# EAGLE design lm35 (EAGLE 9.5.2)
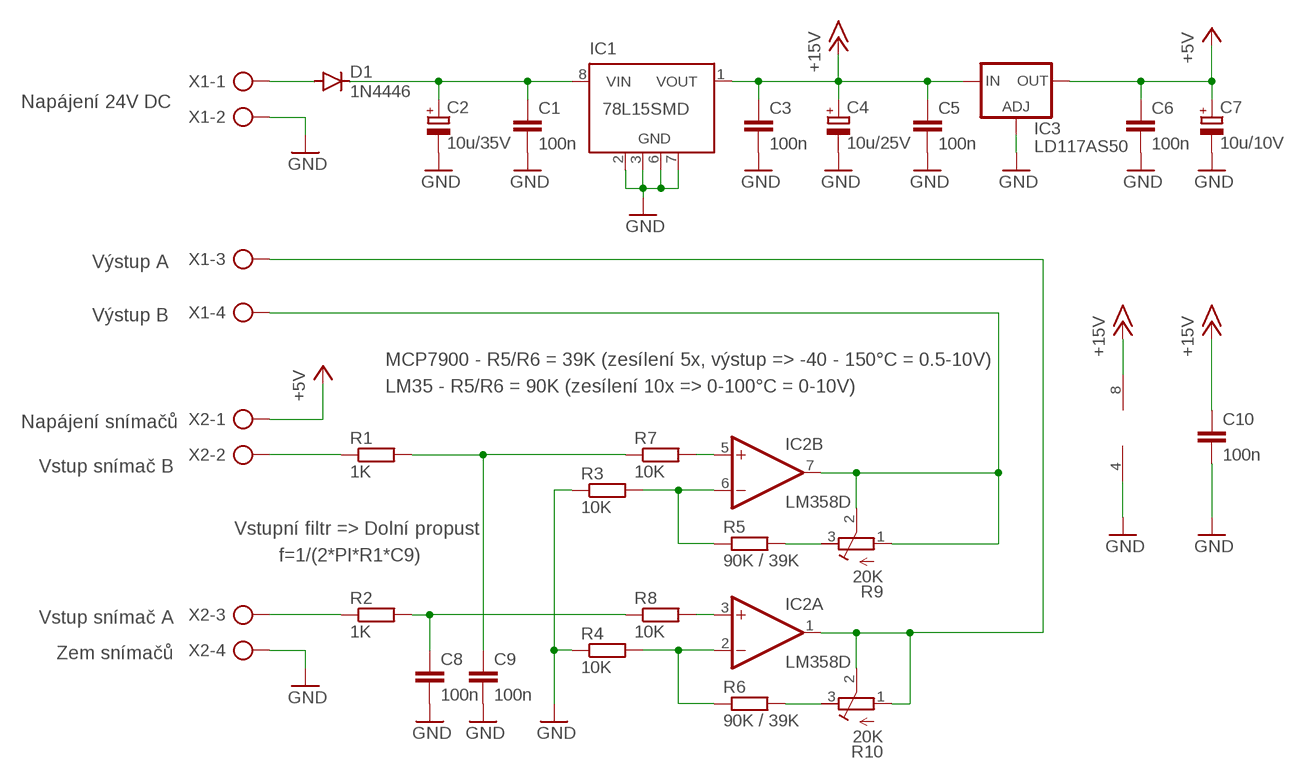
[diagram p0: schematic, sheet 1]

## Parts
C1  100n  C-EUC1206K  [C1206K]
C2  10u/35V  CPOL-EUE2.5-6  [E2,5-6]
C3  100n  C-EUC1206K  [C1206K]
C4  10u/25V  CPOL-EUE2.5-6  [E2,5-6]
C5  100n  C-EUC1206K  [C1206K]
C6  100n  C-EUC1206K  [C1206K]
C7  10u/10V  CPOL-EUE2.5-6  [E2,5-6]
C8  100n  C-EUC1206K  [C1206K]
C9  100n  C-EUC1206K  [C1206K]
C10  100n  C-EUC1206K  [C1206K]
D1  1N4446  [DO35-10]
IC1  78L15SMD  [SO08]
IC2  LM358D  [SO08]
IC3  LD117AS50  LD117AS50TR  [SOT223]
R1  1K  R-EU_M1206  [M1206]
R2  1K  R-EU_M1206  [M1206]
R3  10K  R-EU_M1206  [M1206]
R4  10K  R-EU_M1206  [M1206]
R5  90K / 39K  R-EU_M1206  [M1206]
R6  90K / 39K  R-EU_M1206  [M1206]
R7  10K  R-EU_M1206  [M1206]
R8  10K  R-EU_M1206  [M1206]
R9  20K  R-TRIMM64Y  [RTRIM64Y]
R10  20K  R-TRIMM64Y  [RTRIM64Y]
X1  AK500/4  [AK500/4]
X2  AK500/4  [AK500/4]

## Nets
+5V: C6.1 C7.+ IC3.4(OUT) X2.1
+15V: C3.1 C4.+ C5.1 C10.1 IC1.1(VOUT) IC2.8(P:V+) IC3.3(IN)
GND: C1.2 C2.- C3.2 C4.- C5.2 C6.2 C7.- C8.2 C9.2 C10.2 IC1.2(GND) IC1.3(GND) IC1.6(GND) IC1.7(GND) IC2.4(P:V-) IC3.1(ADJ) R3.1 R4.1 X1.2 X2.4
N$1: D1.A X1.1
N$2: C1.1 C2.+ D1.C IC1.8(VIN)
N$3: R1.1 X2.2
N$4: R2.1 X2.3
N$5: C8.1 R2.2 R8.1
N$6: C9.1 R1.2 R7.1
N$7: IC2.5(B:+IN) R7.2
N$8: IC2.6(B:-IN) R3.2 R5.1
N$9: IC2.3(A:+IN) R8.2
N$10: IC2.2(A:-IN) R4.2 R6.1
N$11: IC2.7(B:OUT) R9.1(A) R9.2(S) X1.4
N$12: IC2.1(A:OUT) R10.1(A) R10.2(S) X1.3
N$13: R6.2 R10.3(E)
N$14: R5.2 R9.3(E)
Unconnected: IC1.4(NC) IC1.5(NC)

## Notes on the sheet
- Napájení 24V DC
- Výstup A
- Výstup B
- MCP7900 - R5/R6 = 39K (zesílení 5x, výstup => -40 - 150°C = 0.5-10V)
- LM35 - R5/R6 = 90K (zesílení 10x => 0-100°C = 0-10V)
- Napájení snímačů
- Vstup snímač B
- Vstupní filtr => Dolní propust
- f=1/(2*PI*R1*C9)
- Vstup snímač A
- Zem snímačů

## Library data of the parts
C1 C3 C5 C6 C8-C10 = rcl:C-EU: CAPACITOR, European symbol; SPICEPREFIX: C
C2 C4 C7 = rcl:CPOL-EU: POLARIZED CAPACITOR, European symbol; SPICEPREFIX: C
D1 = diode:1N4446: DIODE
IC1 = linear:78L*SMD: Positive VOLTAGE REGULATOR
IC2 = linear:LM358: OP AMP also LM158; LM258; LM2904 Source: http://cache.national.com/ds/LM/LM158.pdf
IC3 = v-reg:LD117A?*: Low drop fixed and adjustable positive voltage regulators 1 A Source: http://www.st.com/stonline/products/literature/ds/7194/ld1117axx.pdf
R1-R8 = rcl:R-EU_: RESISTOR, European symbol; SPICEPREFIX: R
R9 R10 = rcl:R-TRIMM: Trimm resistor; SPICEMODEL: X; SPICEPREFIXL: POT
X1 X2 = con-ptr500:AK500/4: CONNECTOR; OC_FARNELL: unknown; OC_NEWARK: unknown

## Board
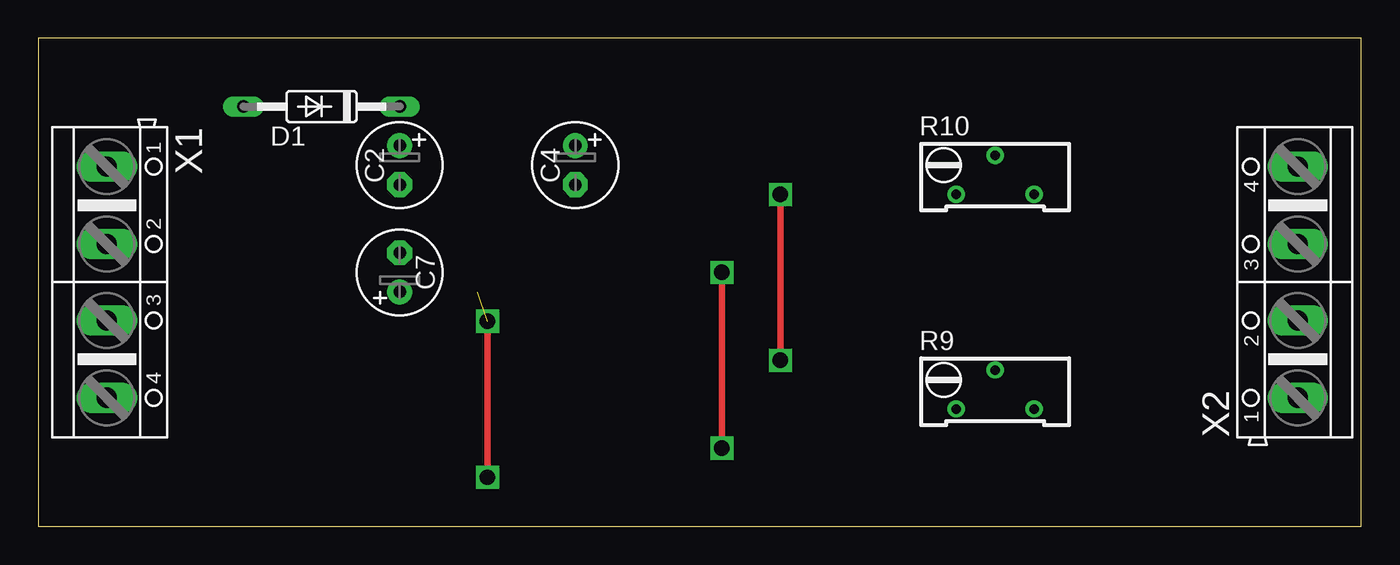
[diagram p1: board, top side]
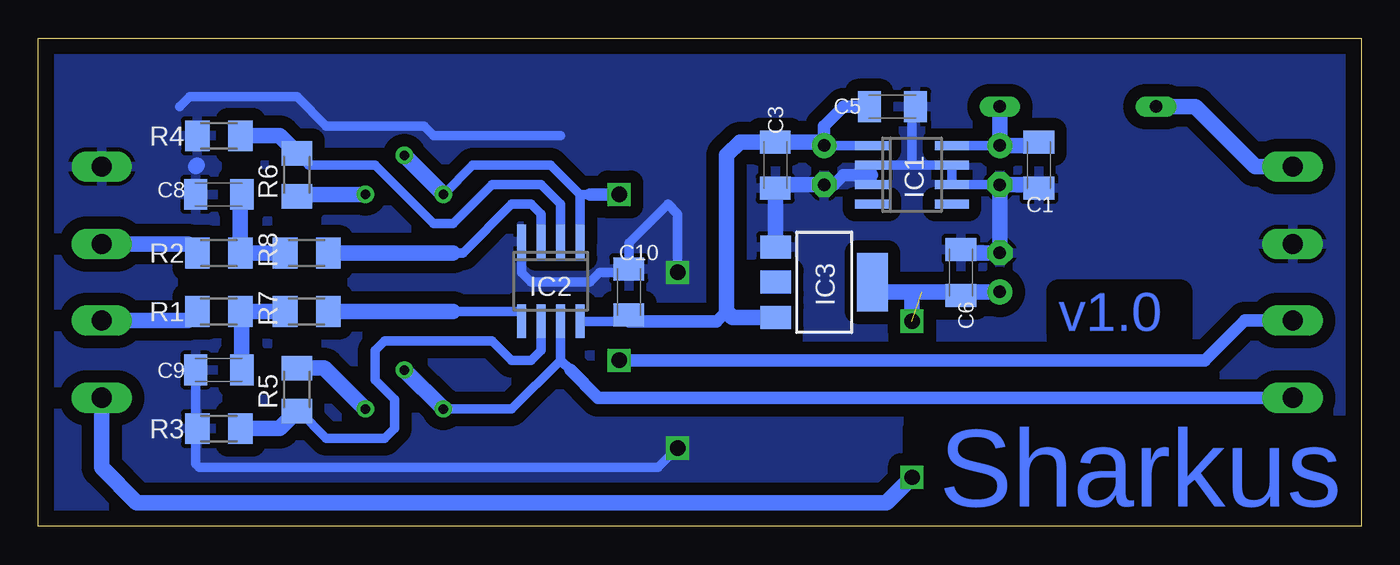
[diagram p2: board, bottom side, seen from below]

Size 86.03 x 31.74 mm. Coordinates in mm from the lower left corner, seen from the top.
Outline: 0,0 86.03,0 86.03,31.74 0,31.74 0,0
Copper layers (1*16): Top 0.035mm / dielectric 1.5mm / Bottom 0.035mm
Design rules "default": minimum track width 6mil, minimum drill 0.35mm, track to track 6mil, track to pad 6mil, pad to pad 6mil, via to via 6mil, smd to smd 6mil, copper to edge 40mil, drill to drill 6mil, minimum pad ring 10mil, minimum via ring 8mil, stop-mask expansion 4mil, vias tented up to drill 0mil, thermal gap 10mil

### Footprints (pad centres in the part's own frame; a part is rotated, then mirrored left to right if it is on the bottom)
C1206K = smd 1.5 x 2: 1 -1.5,0; 2 1.5,0
E2,5-6 = drill 0.813 pad 1.6: + -1.27,0 | drill 0.813 pad 1.6 octagon: - 1.27,0
DO35-10 = drill 0.813 long: A 5.08,0; C -5.08,0
SO08 = smd 0.6 x 2.2: 1 -1.905,-2.6; 2 -0.635,-2.6; 3 0.635,-2.6; 4 1.905,-2.6; 5 1.905,2.6; 6 0.635,2.6; 7 -0.635,2.6; 8 -1.905,2.6
SOT223 = smd 1.5 x 2: 1 -2.3,-3.15; 2 0,-3.15; 3 2.3,-3.15 | smd 3.8 x 2: 4 0,3.15
M1206 = smd 1.6 x 2: 1 -1.4,0; 2 1.4,0
RTRIM64Y = drill 0.61: 1 0,-2.54; 2 -2.54,0; 3 0,2.54
AK500/4 = drill 1.321 long: 1 -7.518,0; 2 -2.489,0; 3 2.489,0; 4 7.518,0

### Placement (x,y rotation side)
C1  20.95,23.5 270 bottom
C2  23.5,23.5 270 top
C3  38.1,23.5 270 bottom
C4  34.92,23.5 270 top
C5  30.48,27.3 0 bottom
C6  26.04,16.51 90 bottom
C7  23.5,16.51 90 top
C8  74.3,21.59 180 bottom
C9  74.3,10.16 180 bottom
C10  47.62,15.24 90 bottom
D1  18.41,27.3 180 top
IC1  29.21,22.86 270 bottom
IC2  52.7,15.94 180 bottom
IC3  34.92,15.88 270 bottom
R1  74.3,13.97 0 bottom
R2  74.3,17.78 0 bottom
R3  74.3,6.35 0 bottom
R4  74.3,25.4 0 bottom
R5  69.22,8.89 90 bottom
R6  69.22,22.86 270 bottom
R7  68.58,13.97 0 bottom
R8  68.58,17.78 0 bottom
R9  62.23,7.62 270 top
R10  62.23,21.59 270 top
X1  4.45,15.88 270 top
X2  81.92,15.88 90 top

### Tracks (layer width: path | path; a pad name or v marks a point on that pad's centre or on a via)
+5V  (via drill 1 pad 1)  (1 unrouted)
  Top 0.406: v29.21,13.34 v29.21,3.17
  Bottom 1.016: C7.+ 25.8,15.24 C6.1 26.27,15.24 29.21,15.24 v29.21,13.34 | IC3.4 31.14,15.24 28.57,15.24 | X2.1 81.92,3.81 79.63,1.52 30.86,1.52 v29.21,3.17
+15V
  Bottom 0.61: IC1.1 C4.+ | IC2.8 48.03,13.34 C10.1
  Bottom 0.813: C5.1 33.66,27.3 34.92,26.04 C4.+ | C10.1 47.62,13.34 41.91,13.34 41.27,13.97
  Bottom 1.016: C4.+ 35.16,25 C3.1 40.41,25 41.27,24.13 41.27,13.97 40.88,13.57 IC3.3
GND  (via drill 1 pad 1)
  Top 0.406: v44.45,5.08 v44.45,16.51
  Bottom 0.61: IC1.3 31.81,22.86 IC1.2 29.21,23.5 | C2.- IC1.6 IC1.7 29.21,23.5 | C5.2 29.21,27.07 29.21,23.5 | 52.07,25.4 60.33,25.4 60.96,26.04 67.31,26.04 69.22,27.94 76.2,27.94 76.83,27.3 | IC2.4 54.61,16.51 53.98,15.88 50.16,15.88 49.53,16.51 47.85,16.51 C10.2 47.62,18.41 45.09,20.95 44.45,20.32 v44.45,16.51 | C9.2 75.8,4.04 75.56,3.81 45.72,3.81 v44.45,5.08
  Bottom 0.813: C4.- 34.29,22.23 33.66,22.86 31.81,22.86
  Bottom 1.016: C6.2 25.8,17.78 C7.- C2.- 21.18,22.23 C1.2 | C4.- 37.87,22.23 C3.2 38.1,18.2 IC3.1 | 75.69,21.69 C8.2 | 75.8,23.39 75.69,23.5
  pour Bottom (isolate 0.813): 0,31.75 85.72,31.75 85.72,0 0,0
N$1
  Bottom 1.016: D1.A 10.79,27.3 6.88,23.39 X1.1
N$2
  Bottom 0.61: IC1.8 C2.+
  Bottom 1.016: C1.1 21.18,24.77 C2.+ D1.C
N$3
  Bottom 1.016: R1.1 76.28,13.39 X2.2
N$4
  Bottom 1.016: R2.1 76.28,18.36 X2.3
N$5
  Bottom 1.016: R8.1 R2.2 72.89,21.49 C8.1
N$6
  Bottom 1.016: R7.1 R1.2 72.8,13.87 C9.1
N$7
  Bottom 0.61: IC2.5 54.61,13.97 59.05,13.97
  Bottom 1.016: 59.05,13.97 R7.2
N$8
  Bottom 0.61: R5.1 69.08,7.49 67.31,5.71 63.5,5.71 62.87,6.35 62.87,8.26 64.14,9.53 64.14,11.43 63.5,12.06 56.52,12.06 55.24,10.79 53.98,10.79 53.34,11.43 IC2.6
  Bottom 1.016: R5.1 70.36,6.35 R3.2
N$9
  Bottom 0.61: IC2.3 53.34,20.32 53.98,20.95 55.24,20.95 58.42,17.78 59.05,17.78
  Bottom 1.016: 59.05,17.78 R8.2
N$10
  Bottom 0.61: R6.1 68.45,23.5 64.14,23.5 60.33,19.68 59.05,19.68 56.52,22.23 53.34,22.23 52.07,20.95 IC2.2
  Bottom 1.016: R6.1 70.36,25.4 R4.2
N$11
  Bottom 0.61: R9.1 55.24,7.62 52.07,10.79 | IC2.7 52.07,10.79 | 51.44,10.16 52.07,10.79
  Bottom 0.813: X1.4 49.63,8.36 51.44,10.16
  Bottom 1.016: R9.1 R9.2
N$12  (via drill 1 pad 1)
  Top 0.406: v48.26,21.59 v48.26,10.79
  Bottom 0.61: IC2.1 50.8,21.59 | 50.8,21.59 52.7,23.5 57.78,23.5 R10.1 | 50.16,21.59 50.8,21.59
  Bottom 0.813: X1.3 7.57,13.39 10.16,10.79 v48.26,10.79 | v48.26,21.59 50.16,21.59
  Bottom 1.016: R10.1 R10.2
N$13
  Bottom 1.016: R6.2 68.71,21.46 68.58,21.59 R10.3
N$14
  Bottom 1.016: R5.2 67.44,10.29 R9.3

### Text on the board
Bottom: v1.0 | Sharkus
